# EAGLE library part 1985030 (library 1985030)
PCB terminal block, nominal current: 8 A, rated voltage (III/2): 250 V, nominal cross section: 1.5 mm?, Number of potentials: 9, Number of rows: 1, Number of positions per row: 9, product range: PTSA 1,5, pitch: 3.5 mm, connection method: Push-in spring connection, mounting: Wave soldering, conductor/PCB connection direction: 45 ?, color: green, Pin layout: Linear pinning, Solder pin [P]: 3.6 mm, type of packaging: packed in cardboard. Soldering legs in front area, one-rowed Source: Datasheet
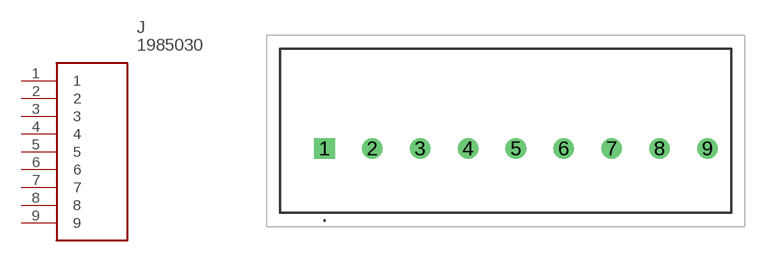
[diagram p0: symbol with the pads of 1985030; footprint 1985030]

Designator prefix J

## 1985030 (Description: PCB terminal block, nominal current: 8 A, rated voltage (III/2): 250 V, nominal cross section: 1.5 mm?, Number of potentials: 9, Number of rows: 1, Number of positions per row: 9, product range: PTSA 1,5, pitch: 3.5 mm, connection method: Push-in spring connection, mounting: Wave soldering, conductor/PCB connection direction: 45 ?, color: green, Pin layout: Linear pinning, Solder pin [P]: 3.6 mm, type of packaging: packed in cardboard. Soldering legs in front area, one-rowed; Height: 13.1mm; Manufacturer_Name: Phoenix Contact; Manufacturer_Part_Number: 1985030)  [1985030]
1  1
2  2
3  3
4  4
5  5
6  6
7  7
8  8
9  9

## Footprint 1985030 (pad centres in mm)
1985030
drill 1 pad 1.5 square: 1 0,0
drill 1 pad 1.5: 2 3.5,0; 3 7,0; 4 10.5,0; 5 14,0; 6 17.5,0; 7 21,0; 8 24.5,0; 9 28,0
